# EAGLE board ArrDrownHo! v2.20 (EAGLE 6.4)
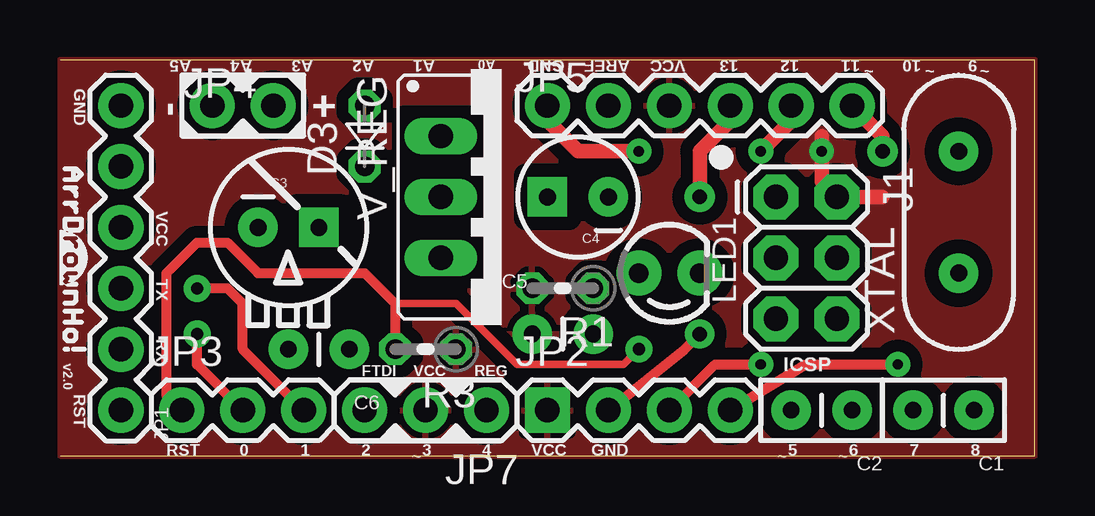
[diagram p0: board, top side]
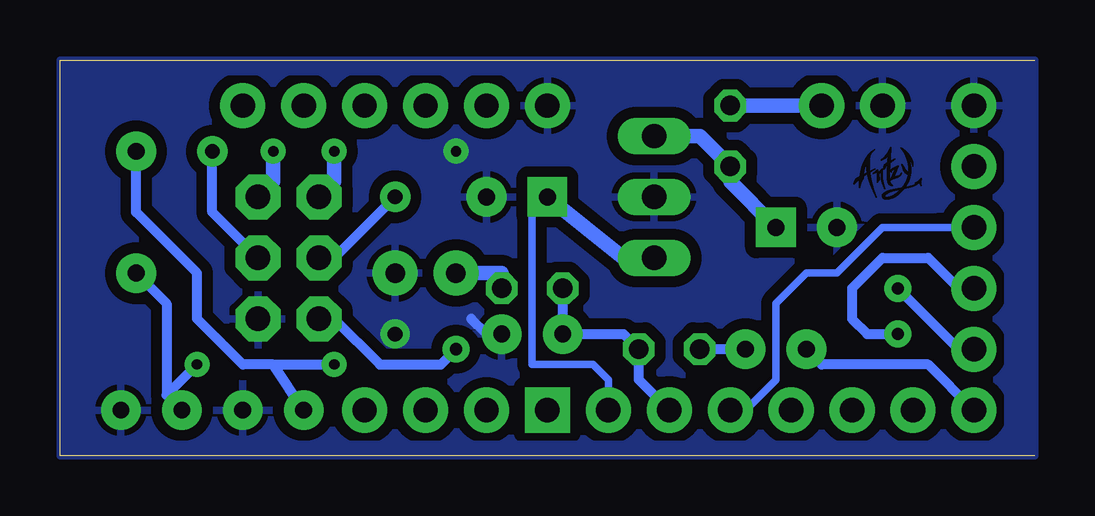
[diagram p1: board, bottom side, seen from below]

Size 40.64 x 16.51 mm. Coordinates in mm from the lower left corner, seen from the top.
Outline: 0,0 40.64,0 40.64,16.51 0,16.51
Copper layers (1*16): Top 0.035mm / dielectric 1.5mm / Bottom 0.035mm
Design rules "default *": minimum track width 16mil, minimum drill 24mil, track to track 8mil, track to pad 8mil, pad to pad 8mil, via to via 8mil, smd to smd 8mil, copper to edge 0mil, drill to drill 8mil, minimum pad ring 10mil, minimum via ring 12mil, stop-mask expansion 4mil, vias tented up to drill 0mil, thermal gap 10mil
Holes 0.51 mm at -3.17,-3.81 44.45,20.32 44.45,-3.81 20.64,20.32 20.64,-3.81 -3.17,20.32
tRestrict: area 11.8,1 to 13.6,2.8; area 16.9,1 to 18.7,2.8; area 1.6,13.7 to 3.4,15.5; area 1.6,11.2 to 3.4,13; area 1.6,8.6 to 3.4,10.4; area 1.6,6.1 to 3.4,7.9; area 1.6,3.5 to 3.4,5.3; area 1.6,1 to 3.4,2.8; area 31.5,7.4 to 33.3,9.2; area 31.5,9.9 to 33.3,11.7; area 28.9,9.9 to 30.7,11.7; area 28.9,4.8 to 30.7,6.6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
bRestrict: area 22,13.7 to 23.8,15.5; area 24.5,13.7 to 26.3,15.5; area 27,13.7 to 28.8,15.5; area 29.6,13.7 to 31.4,15.5; area 32.1,13.7 to 33.9,15.5; area 27,1 to 28.8,2.8; area 24.5,1 to 26.3,2.8; area 22,1 to 23.8,2.8; area 9.3,1 to 11.1,2.8; area 6.7,1 to 8.5,2.8; area 4.2,1 to 6,2.8; area 19.4,1 to 21.2,2.8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

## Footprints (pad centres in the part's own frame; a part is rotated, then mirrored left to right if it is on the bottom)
CAP-PTH-SMALLEZ = drill 0.7 pad 1.651: 1 0,0; 2 2.54,0
CPOL-RADIAL-100UF-25V = drill 0.7 pad 1.651 square: 1 1.27,0 | drill 0.7 pad 1.651: 2 -1.27,0
CPOL-RADIAL-10UF-25V = drill 0.7 pad 1.651 square: 1 1.27,0 | drill 0.7 pad 1.651: 2 -1.27,0
CAP-PTH-SMALL = drill 0.7 pad 1.651: 1 0,0; 2 2.54,0
D-2.5 = drill 0.813 octagon: A 1.27,0; C -1.27,0
2X3 = drill 1.016 pad 1.88 octagon: 1 0,0; 2 0,2.54; 3 2.54,0; 4 2.54,2.54; 5 5.08,0; 6 5.08,2.54
1X06 = drill 1.016 pad 1.88: 1 0,0; 2 2.54,0; 3 5.08,0; 4 7.62,0; 5 10.16,0; 6 12.7,0
1X04 = drill 1.016 pad 1.88 square: 1 0,0 | drill 1.016 pad 1.88: 2 2.54,0; 3 5.08,0; 4 7.62,0
1X03 = drill 1.016 pad 1.88: 1 0,0; 2 2.54,0; 3 5.08,0
1X02 = drill 1.016 pad 1.88: 1 0,0; 2 2.54,0
LED3MM = drill 0.813 pad 1.88: A -1.27,0; K 1.27,0
0204V = drill 0.813 octagon: 1 -1.27,0; 2 1.27,0
78XXS = drill 1.016 long: GND 0,-2.54; IN -2.54,-2.54; OUT 2.54,-2.54
HC49US = drill 0.7 pad 1.651: 1 -2.54,0; 2 2.54,0

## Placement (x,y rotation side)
C1  22uF  [CAP-PTH-SMALLEZ]  38.1,1.91 180 top
C2  22uF  [CAP-PTH-SMALLEZ]  33.02,1.91 180 top
C3  100uF  [CPOL-RADIAL-100UF-25V]  9.53,9.53 0 top
C4  10uF  [CPOL-RADIAL-10UF-25V]  21.59,10.79 180 top
C5  0.1uF  [CAP-PTH-SMALL]  19.68,5.08 0 top
C6  0.1uF  [CAP-PTH-SMALL]  12.06,4.45 180 top
D3  1N4001  [D-2.5]  12.7,13.34 90 top
J1  ISP  [2X3]  29.84,10.79 270 top
JP1  SERIAL  [1X06]  2.54,1.91 90 top
JP2  [1X04]  20.32,1.91 0 top
JP3  [1X03]  5.08,1.91 0 top
JP4  9V  [1X02]  6.35,14.61 0 top
JP5  [1X06]  20.32,14.61 0 top
JP7  PWR SEL  [1X03]  17.78,1.91 180 top
LED1  Green  [LED3MM]  25.4,7.62 0 top
R1  1K  [0204V]  20.95,6.99 180 top
R3  10K  [0204V]  15.24,4.45 180 top
V_REG  LM7805  [78XXS]  18.41,10.79 270 top
XTAL  16MHz  [HC49US]  37.47,10.16 90 top

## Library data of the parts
C1 C2 = SparkFun-Capacitors
C3-C6 JP4 JP7 = SparkFun-Passives
D3 = diode
J1 JP1-JP3 JP5 = SparkFun-Connectors
LED1 = SparkFun-LED
R1 R3 = resistor
V_REG = v-reg
XTAL = SparkFun-FreqCtrl

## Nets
5V_REG: C4.1 JP7.1 V_REG.OUT
9V: D3.A JP4.2
AREF: JP5.2
GND: C1.1 C2.1 C3.2 C4.2 C5.2 J1.6 JP1.6 JP2.2 JP4.1 JP5.1 LED1.K V_REG.GND
MISO: J1.1 JP5.5
MOSI: J1.4 JP5.6
N$1: C1.2 JP2.4 XTAL.1
N$2: C2.2 JP2.3 XTAL.2
N$3: JP1.4 JP7.3
N$4: C6.2 JP1.1
N$5: LED1.A R1.1
N$13: C3.1 D3.C V_REG.IN
RST: C6.1 J1.5 JP3.1 R3.2
RX: JP1.3 JP3.2
SCK: J1.3 JP5.4
TX: JP1.2 JP3.3
VCC: C5.1 J1.2 JP2.1 JP5.3 JP7.2 R1.2 R3.1

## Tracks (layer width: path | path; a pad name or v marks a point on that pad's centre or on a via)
5V_REG
  Bottom 0.305: C4.1 20.95,10.16 20.95,3.81 18.41,3.81 17.78,3.17 JP7.1
  Bottom 0.61: C4.1 17.14,8.26 V_REG.OUT
9V
  Bottom 0.61: D3.A JP4.2
GND  (via drill 0.43 pad 0.94, 0.61)
  Top 0.406: JP2.2 26.04,4.45 v26.67,5.08
  Top 0.61: v24.13,12.7 21.59,12.7 20.32,13.97 JP5.1
  Bottom 0.406: C5.2 22.86,5.08 23.5,5.71
  pour Bottom (isolate 0.457): 0,16.51 0,0 40.64,0 40.64,16.51
  pour Bottom (rank 2): 0,0.64 40.64,0.64 40.64,0 0,0
  pour Bottom (rank 2): 0,16.51 40.64,16.51 40.64,15.88 0,15.88
  pour Bottom (rank 2): 0,16.51 0,0 1.27,0 1.27,16.51
  pour Bottom (isolate 0.025, no thermals): 4.1,10.13 6.48,10.13 6.71,10.05 7,9.74 7.21,9.79 7.25,9.93 7.35,10.12 7.52,10.33 7.72,10.46 7.91,10.55 8.08,10.6 8.05,12.06 7.29,13.84 7.06,13.64 6.88,13.53 6.65,13.45 6.58,13.44 6.08,13.44 5.83,13.53 5.63,13.65 5.46,13.8 3.98,12.4
MISO  (via drill 0.43 pad 0.94)
  Top 0.61: v29.21,12.7 30.48,13.97 JP5.5
  Bottom 0.61: J1.1 29.21,11.43 v29.21,12.7
MOSI  (via drill 0.61 pad 1.27)
  Top 0.61: JP5.6 34.29,13.34 v34.29,12.7
  Bottom 0.406: J1.4 34.29,10.16 v34.29,12.7
N$1  (via drill 0.43 pad 0.94)
  Top 0.406: JP2.4 31.11,3.81 v34.92,3.81
  Bottom 0.406: 36.2,2.54 36.2,6.35 XTAL.1 | 36.2,2.54 C1.2 | v34.92,3.81 36.2,2.54
N$2  (via drill 0.43 pad 0.94)
  Top 0.406: JP2.3 27.3,3.81 v29.21,3.81
  Bottom 0.406: 31.75,3.81 C2.2 | 31.75,3.81 v29.21,3.81 | 31.75,3.81 33.02,3.81 34.92,5.71 34.92,7.62 37.47,10.16 XTAL.2
N$3
  Bottom 0.305: JP1.4 6.35,9.53 8.26,7.62 9.53,7.62 10.79,6.35 10.79,3.17 12.06,1.91 JP7.3
N$4
  Bottom 0.406: JP1.1 4.45,3.81 8.89,3.81 C6.2
N$5
  Bottom 0.61: LED1.A 22.23,7.62 R1.1
N$7  (via drill 0.51)
  other vias: -3.17,-3.81
N$8  (via drill 0.51)
  other vias: -3.17,20.32
N$9  (via drill 0.51)
  other vias: 44.45,20.32
N$10  (via drill 0.51)
  other vias: 44.45,-3.81
N$11  (via drill 0.51)
  other vias: 20.64,-3.81
N$13
  Bottom 0.61: V_REG.IN 13.97,13.34 D3.C 12.7,11.43 C3.1
N$17  (via drill 0.51)
  other vias: 20.64,20.32
RST  (via drill 0.51)
  Top 0.305: v24.13,4.45 23.5,3.81 19.05,3.81 16.51,6.35 13.97,6.35
  Top 0.406: JP3.1 4.45,2.54 4.45,7.62 5.71,8.89 6.99,8.89 8.26,7.62 12.7,7.62 13.97,6.35 R3.2
  Bottom 0.406: J1.5 29.21,5.71 27.3,3.81 24.77,3.81 v24.13,4.45 | C6.1 R3.2
RX  (via drill 0.51)
  Top 0.406: JP3.2 5.71,3.81 v5.71,5.08
  Bottom 0.406: JP1.3 3.17,6.99 4.45,8.26 6.35,8.26 7.62,6.99 7.62,5.71 6.99,5.08 v5.71,5.08
SCK  (via drill 0.61 pad 1.27)
  Top 0.61: JP5.4 27.94,13.97 26.67,12.7 v26.67,10.79
  Bottom 0.406: v26.67,10.79 29.21,8.26 J1.3
TX  (via drill 0.51)
  Top 0.406: JP3.3 7.62,4.45 7.62,6.35 6.99,6.99 v5.71,6.99
  Bottom 0.406: JP1.2 3.17,4.45 v5.71,6.99
VCC  (via drill 0.43 pad 0.94)
  Top 0.61: 31.75,13.34 v31.75,12.7 31.75,11.43 J1.2 34.29,10.79
  Bottom 0.406: R1.2 C5.1 17.14,5.08 R3.1 16.51,3.17 JP7.2
  Bottom 0.61: J1.2 31.75,11.43 v31.75,12.7
  pour Top (isolate 0.508): 0,16.51 0,0 40.64,0 40.64,16.51

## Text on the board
tPlace: A5 | A4 | A3 | A2 | A1 | A0 | GND | AREF | VCC | 13 | 12 | 11 | ~ | 10 | ~ | 9 | ~ | GND | - | + | VCC | TX | v2.0 | RX | ICSP | FTDI | VCC | REG | RST | RST | 0 | 1 | 2 | ~ | 3 | 4 | VCC | GND | ~ | 5 | ~ | 6 | 7 | 8
200bmp: ArrDrownHo!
